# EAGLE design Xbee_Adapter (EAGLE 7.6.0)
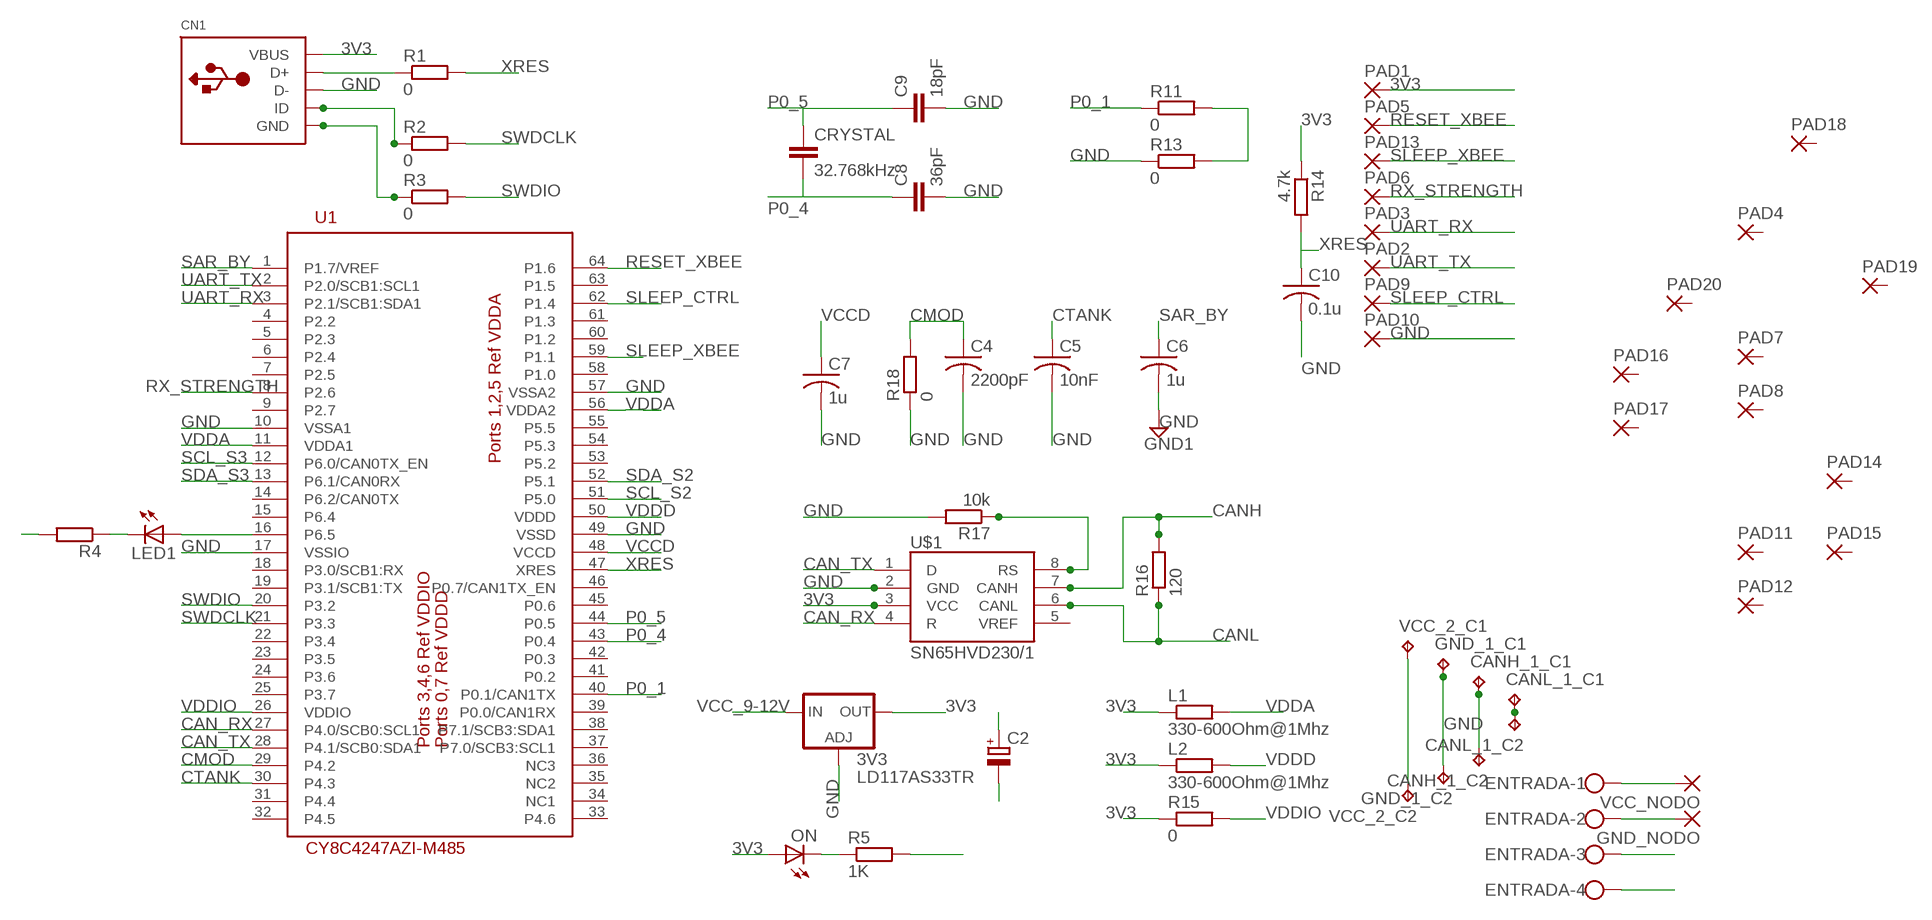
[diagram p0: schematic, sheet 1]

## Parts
3V3  LD117AS33TR  [SOT223]
C2  CPOL-EUA  [PANASONIC_A]
C4  2200pF  C-USC0805  [C0805]
C5  10nF  C-USC0805  [C0805]
C6  1u  C-USC0805  [C0805]
C7  1u  C-USC0805  [C0805]
C8  36pF  C-EUC0805  [C0805]
C9  18pF  C-EUC0805  [C0805]
C10  0.1u  C-USC0805  [C0805]
CANH_1_C1  TPB2,54  [B2,54]
CANH_1_C2  TPB2,54  [B2,54]
CANL_1_C1  TPB2,54  [B2,54]
CANL_1_C2  TPB2,54  [B2,54]
CN1  USBMINIB  [USB-MINIB]
CRYSTAL  32.768kHz  C-EUC0603  [C0603]
ENTRADA  W237-4  [W237-4]
GND_1_C1  TPB2,54  [B2,54]
GND_1_C2  TPB2,54  [B2,54]
GND_NODO  SMD5  [SMD2,54-5,08]
L1  330-600Ohm@1Mhz  R-EU_R0805  [R0805]
L2  330-600Ohm@1Mhz  R-EU_R0805  [R0805]
LED1  LEDCHIP-LED0805  [CHIP-LED0805]
ON  LEDCHIP-LED0805  [CHIP-LED0805]
PAD1  SMD5  [SMD2,54-5,08]
PAD2  SMD5  [SMD2,54-5,08]
PAD3  SMD5  [SMD2,54-5,08]
PAD4  SMD5  [SMD2,54-5,08]
PAD5  SMD5  [SMD2,54-5,08]
PAD6  SMD5  [SMD2,54-5,08]
PAD7  SMD5  [SMD2,54-5,08]
PAD8  SMD5  [SMD2,54-5,08]
PAD9  SMD5  [SMD2,54-5,08]
PAD10  SMD5  [SMD2,54-5,08]
PAD11  SMD5  [SMD2,54-5,08]
PAD12  SMD5  [SMD2,54-5,08]
PAD13  SMD5  [SMD2,54-5,08]
PAD14  SMD5  [SMD2,54-5,08]
PAD15  SMD5  [SMD2,54-5,08]
PAD16  SMD5  [SMD2,54-5,08]
PAD17  SMD5  [SMD2,54-5,08]
PAD18  SMD5  [SMD2,54-5,08]
PAD19  SMD5  [SMD2,54-5,08]
PAD20  SMD5  [SMD2,54-5,08]
R1  0  R-EU_R0805  [R0805]
R2  0  R-EU_R0805  [R0805]
R3  0  R-EU_R0805  [R0805]
R4  R-EU_R0805  [R0805]
R5  1K  R-EU_R0805  [R0805]
R11  0  R-EU_R0805  [R0805]
R13  0  R-EU_R0805  [R0805]
R14  4.7k  R-EU_R0805  [R0805]
R15  0  R-EU_R0805  [R0805]
R16  120  R-EU_R0805  [R0805]
R17  10k  R-EU_R0805  [R0805]
R18  0  R-EU_R0805  [R0805]
U1  CY8C4247AZI-M485  [TQFP64-10X10]
U$1  SN65HVD230/1  [SO8]
VCC_2_C1  TPB2,54  [B2,54]
VCC_2_C2  TPB2,54  [B2,54]
VCC_NODO  SMD5  [SMD2,54-5,08]

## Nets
3V3: 3V3.4(OUT) C2.+ CN1.VBUS L1.1 L2.1 ON.A PAD1.1(P) R14.1 R15.1 U$1.3(VCC)
CAN_RX: U1.27(P4.0/SCB0:SCL1) U$1.4(R)
CAN_TX: U1.28(P4.1/SCB0:SDA1) U$1.1(D)
CANH: CANH_1_C1.TP CANH_1_C2.TP ENTRADA.3 R16.2 U$1.7(CANH)
CANL: CANL_1_C1.TP CANL_1_C2.TP ENTRADA.4 R16.1 U$1.6(CANL)
CMOD: C4.1 R18.2 U1.29(P4.2)
CTANK: C5.1 U1.30(P4.3)
GND: 3V3.1(ADJ) C2.- C4.2 C5.2 C6.2 C7.2 C8.2 C9.2 C10.2 CN1.D- ENTRADA.2 GND_1_C1.TP GND_1_C2.TP GND_NODO.1(P) PAD10.1(P) R4.2 R5.2 R13.1 R17.2 R18.1 U1.10(VSSA1) U1.17(VSSIO) U1.49(VSSD) U1.57(VSSA2) U$1.2(GND) ; supply symbol labelled GND1
N$1: CN1.D+ R1.1
N$2: CN1.ID R2.1
N$3: CN1.GND R3.1
N$4: R11.2 R13.2
N$5: LED1.A U1.16(P6.5)
N$6: LED1.C R4.1
N$9: R17.1 U$1.8(RS)
N$10: ON.C R5.1
P0_1: R11.1 U1.40(P0.1/CAN1TX)
P0_4: C8.1 CRYSTAL.2 U1.43(P0.4)
P0_5: C9.1 CRYSTAL.1 U1.44(P0.5)
RESET_XBEE: PAD5.1(P) U1.64(P1.6)
RX_STRENGTH: PAD6.1(P) U1.8(P2.6)
SAR_BY: C6.1 U1.1(P1.7/VREF)
SCL_S2: U1.51(P5.0)
SCL_S3: U1.12(P6.0/CAN0TX_EN)
SDA_S2: U1.52(P5.1)
SDA_S3: U1.13(P6.1/CAN0RX)
SLEEP_CTRL: PAD9.1(P) U1.62(P1.4)
SLEEP_XBEE: PAD13.1(P) U1.59(P1.1)
SWDCLK: R2.2 U1.21(P3.3)
SWDIO: R3.2 U1.20(P3.2)
UART_RX: PAD3.1(P) U1.3(P2.1/SCB1:SDA1)
UART_TX: PAD2.1(P) U1.2(P2.0/SCB1:SCL1)
VCC_9-12V: 3V3.3(IN) ENTRADA.1 VCC_2_C1.TP VCC_2_C2.TP VCC_NODO.1(P)
VCCD: C7.1 U1.48(VCCD)
VDDA: L1.2 U1.11(VDDA1) U1.56(VDDA2)
VDDD: L2.2 U1.50(VDDD)
VDDIO: R15.2 U1.26(VDDIO)
XRES: C10.1 R1.2 R14.2 U1.47(XRES)
Unconnected: PAD4.1(P) PAD7.1(P) PAD8.1(P) PAD11.1(P) PAD12.1(P) PAD14.1(P) PAD15.1(P) PAD16.1(P) PAD17.1(P) PAD18.1(P) PAD19.1(P) PAD20.1(P) U1.4(P2.2) U1.5(P2.3) U1.6(P2.4) U1.7(P2.5) U1.9(P2.7) U1.14(P6.2/CAN0TX) U1.15(P6.4) U1.18(P3.0/SCB1:RX) U1.19(P3.1/SCB1:TX) U1.22(P3.4) U1.23(P3.5) U1.24(P3.6) U1.25(P3.7) U1.31(P4.4) U1.32(P4.5) U1.33(P4.6) U1.34(NC1) U1.35(NC2) U1.36(NC3) U1.37(P7.0/SCB3:SCL1) U1.38(P7.1/SCB3:SDA1) U1.39(P0.0/CAN1RX) U1.41(P0.2) U1.42(P0.3) U1.45(P0.6) U1.46(P0.7/CAN1TX_EN) U1.53(P5.2) U1.54(P5.3) U1.55(P5.5) U1.58(P1.0) U1.60(P1.2) U1.61(P1.3) U1.63(P1.5) U$1.5(VREF)

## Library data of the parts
3V3 = v-reg:LD117A?*: Low drop fixed and adjustable positive voltage regulators 1 A Source: http://www.st.com/stonline/products/literature/ds/7194/ld1117axx.pdf
C2 = rcl:CPOL-EU: POLARIZED CAPACITOR, European symbol
C4-C7 C10 = rcl:C-US: CAPACITOR, American symbol
C8 C9 CRYSTAL = rcl:C-EU: CAPACITOR, European symbol
CANH_1_C1 CANH_1_C2 CANL_1_C1 CANL_1_C2 GND_1_C1 GND_1_C2 VCC_2_C1 VCC_2_C2 = testpad:TP: Test pad
CN1 = adafruit:USB: USB Connectors USBMINIB - Surface Mount Female Mini-B USB Connector 4UConnector: 06564 By microbuilder.eu Thru-hole RA Female Mini-B USB Connector 4UConnector: 18732 By ladyada.net
ENTRADA = con-wago-500:W237-4: WAGO SCREW CLAMP; OC_FARNELL: unknown; OC_NEWARK: unknown
GND_NODO PAD1-PAD20 VCC_NODO = wirepad:SMD5: SMD PAD
L1 L2 R1-R5 R11 R13-R18 = rcl:R-EU_: RESISTOR, European symbol
LED1 ON = adafruit:LED: LED
U1 = CypressPSoC:CY8C4247AZI-M485
U$1 = texas_instruments:SN65HVD230/1

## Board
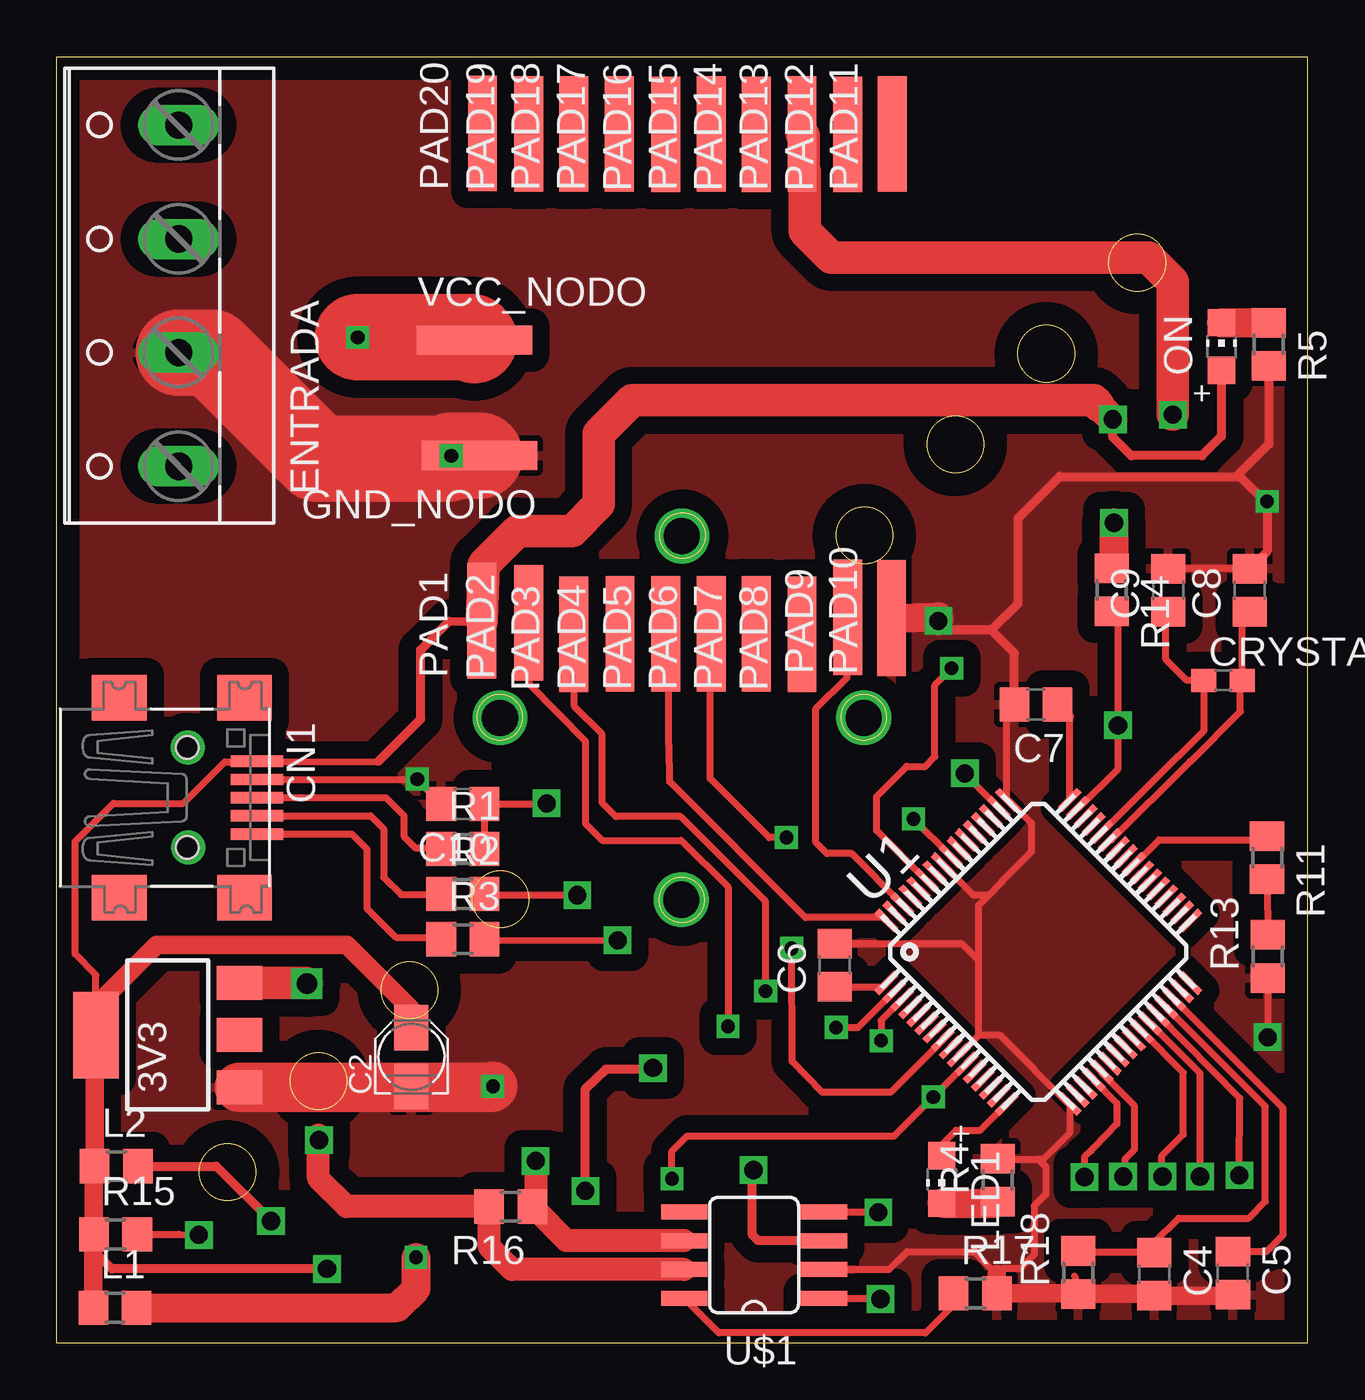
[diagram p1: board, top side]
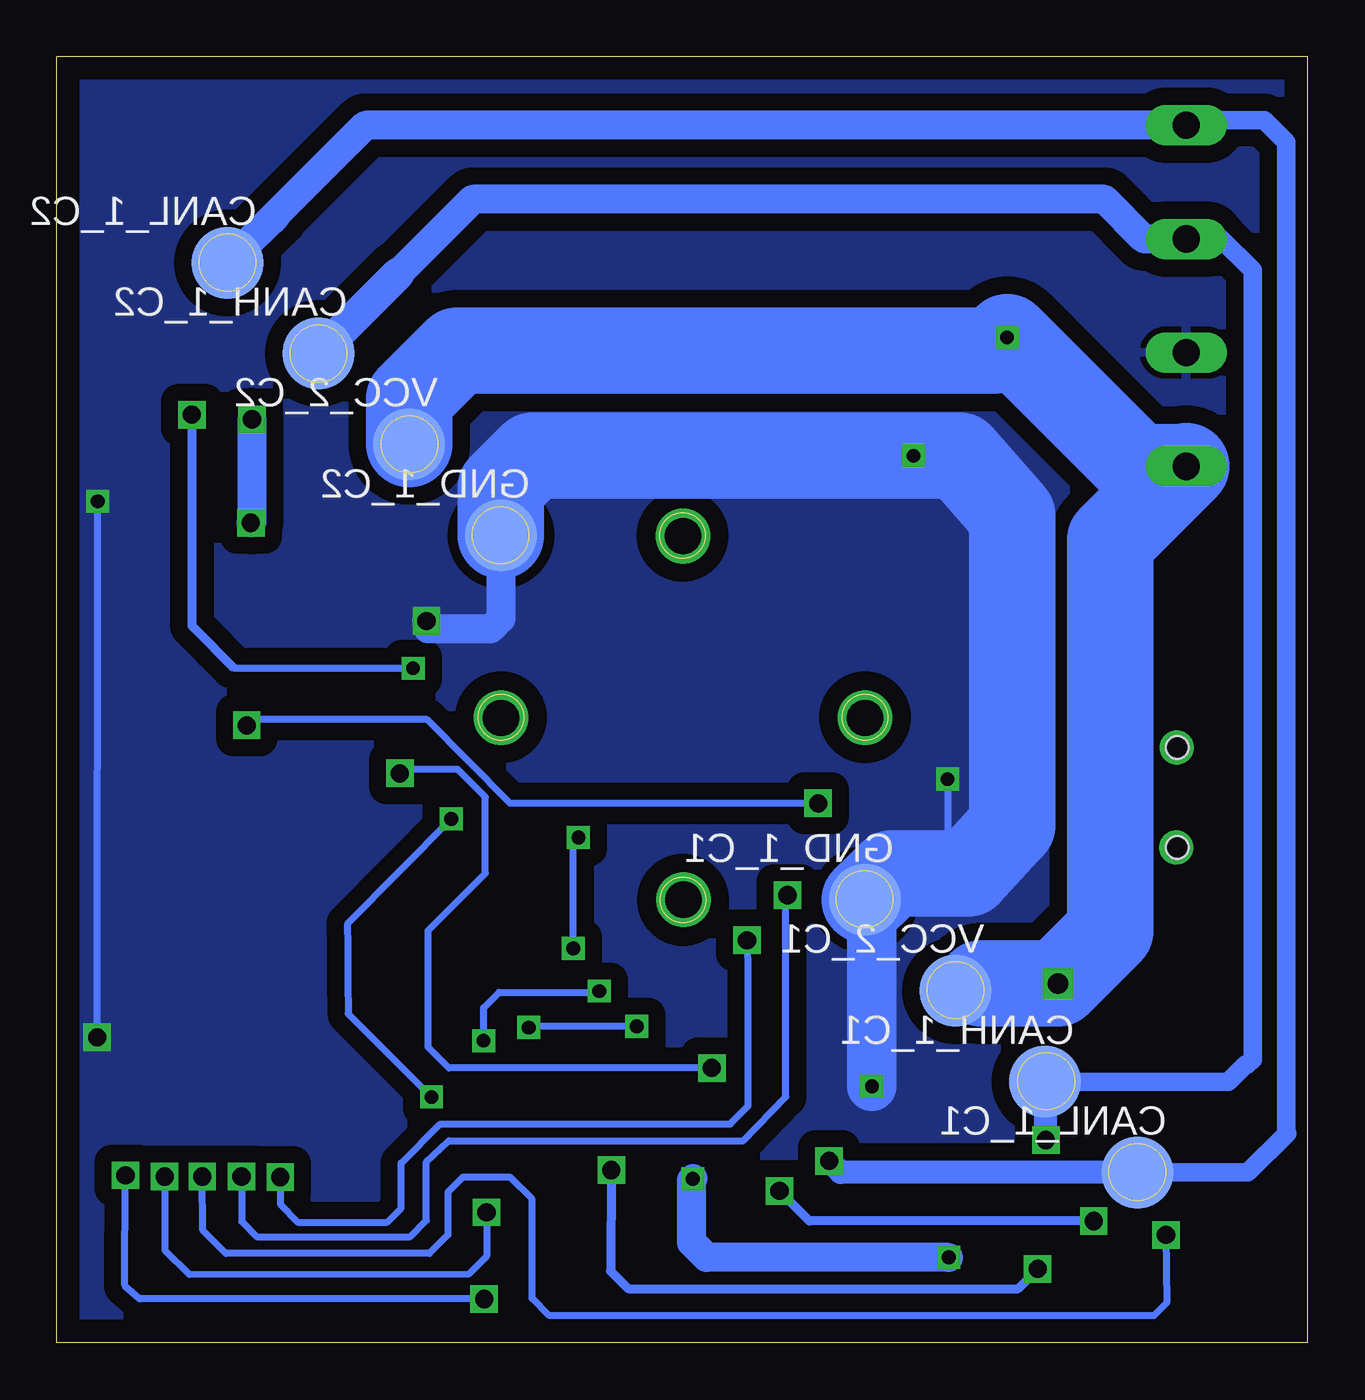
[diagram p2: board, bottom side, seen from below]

Size 55 x 56.55 mm. Coordinates in mm from the lower left corner, seen from the top.
Outline: 0,0 0,56.55 55,56.55 55,0 0,0
Outline: circle at 27.47,19.47 radius 1
Outline: circle at 19.47,27.5 radius 1
Outline: circle at 35.47,27.5 radius 1
Outline: circle at 43.5,43.5 radius 1.25
Outline: circle at 47.5,47.5 radius 1.25
Outline: circle at 43.5,43.5 radius 1.25
Outline: circle at 39.5,39.5 radius 1.25
Outline: circle at 35.5,35.5 radius 1.25
Outline: circle at 15.5,15.5 radius 1.25
Outline: circle at 11.5,11.5 radius 1.25
Outline: circle at 47.5,47.5 radius 1.25
Outline: circle at 39.5,39.5 radius 1.25
Outline: circle at 19.5,19.5 radius 1.25
Outline: circle at 7.5,7.5 radius 1.25
Outline: circle at 19.5,19.5 radius 1.25
Outline: circle at 15.5,15.5 radius 1.25
Outline: circle at 11.5,11.5 radius 1.25
Outline: circle at 35.5,35.5 radius 1.25
Outline: circle at 27.5,35.5 radius 1
Outline: circle at 7.5,7.5 radius 1.25
Copper layers (1*16): Top 0.035mm / dielectric 1.5mm / Bottom 0.035mm
Design rules "default": minimum track width 10mil, minimum drill 24mil, track to track 8mil, track to pad 8mil, pad to pad 8mil, via to via 8mil, smd to smd 8mil, copper to edge 40mil, drill to drill 8mil, minimum pad ring 10mil, minimum via ring 8mil, stop-mask expansion 4mil, vias tented up to drill 0mil, thermal gap 10mil

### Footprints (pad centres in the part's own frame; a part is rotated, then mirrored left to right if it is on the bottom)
SOT223 = smd 1.5 x 2: 1 -2.3,-3.15; 2 0,-3.15; 3 2.3,-3.15 | smd 3.8 x 2: 4 0,3.15
PANASONIC_A = smd 2 x 1.5: + 1.3,0; - -1.3,0
C0805 = smd 1.3 x 1.5: 1 -0.95,0; 2 0.95,0
B2,54 = smd 3.175 x 3.175 bottom: P$1 0,0 | smd 2.54 x 2.54 bottom: TP 0,0
USB-MINIB = smd 0.5 x 2.308: D+ 0,4.064; D- -0.8,4.064; GND 1.6,4.064; ID 0.8,4.064; VBUS -1.6,4.064 | smd 2 x 2.4: GND1 -4.4,-2; GND2 -4.4,3.5; GND3 4.4,3.5; GND4 4.4,-2 | hole 1: -2.2,1; 2.2,1
C0603 = smd 1.1 x 1: 1 -0.85,0; 2 0.85,0
W237-4 = drill 1.194 long: 1 -7.5,-1.27; 2 -2.5,-1.27; 3 2.5,-1.27; 4 7.5,-1.27
SMD2,54-5,08 = smd 1.27 x 5.08: 1 0,0
R0805 = smd 1.3 x 1.5: 1 -0.95,0; 2 0.95,0
CHIP-LED0805 = smd 1.2 x 1.2: A 0,-1.05; C 0,1.05
TQFP64-10X10 = smd 1.2 x 0.3: 1 -5.7,3.75; 2 -5.7,3.25; 3 -5.7,2.75; 4 -5.7,2.25; 5 -5.7,1.75; 6 -5.7,1.25; 7 -5.7,0.75; 8 -5.7,0.25; 9 -5.7,-0.25; 10 -5.7,-0.75; 11 -5.7,-1.25; 12 -5.7,-1.75; 13 -5.7,-2.25; 14 -5.7,-2.75; 15 -5.7,-3.25; 16 -5.7,-3.75; 33 5.7,-3.75; 34 5.7,-3.25; 35 5.7,-2.75; 36 5.7,-2.25; 37 5.7,-1.75; 38 5.7,-1.25; 39 5.7,-0.75; 40 5.7,-0.25; 41 5.7,0.25; 42 5.7,0.75; 43 5.7,1.25; 44 5.7,1.75; 45 5.7,2.25; 46 5.7,2.75; 47 5.7,3.25; 48 5.7,3.75 | smd 0.3 x 1.2: 17 -3.75,-5.7; 18 -3.25,-5.7; 19 -2.75,-5.7; 20 -2.25,-5.7; 21 -1.75,-5.7; 22 -1.25,-5.7; 23 -0.75,-5.7; 24 -0.25,-5.7; 25 0.25,-5.7; 26 0.75,-5.7; 27 1.25,-5.7; 28 1.75,-5.7; 29 2.25,-5.7; 30 2.75,-5.7; 31 3.25,-5.7; 32 3.75,-5.7; 49 3.75,5.7; 50 3.25,5.7; 51 2.75,5.7; 52 2.25,5.7; 53 1.75,5.7; 54 1.25,5.7; 55 0.75,5.7; 56 0.25,5.7; 57 -0.25,5.7; 58 -0.75,5.7; 59 -1.25,5.7; 60 -1.75,5.7; 61 -2.25,5.7; 62 -2.75,5.7; 63 -3.25,5.7; 64 -3.75,5.7
SO8 = smd 0.66 x 2.032: 1 -1.905,-3.073; 2 -0.635,-3.073; 3 0.635,-3.073; 4 1.905,-3.073; 5 1.905,3.073; 6 0.635,3.073; 7 -0.635,3.073; 8 -1.905,3.073

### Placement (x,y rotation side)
3V3  4.87,13.53 90 top
C2  15.59,12.56 90 top
C4  48.25,3.01 270 top
C5  51.71,3.07 270 top
C6  34.21,16.6 90 top
C7  43.04,28.06 180 top
C8  52.44,33.09 90 top
C9  48.86,33.09 90 top
C10  17.85,23.69 180 top
CANH_1_C1  11.55,11.47 0 top
CANH_1_C2  43.5,43.5 0 top
CANL_1_C1  7.48,7.48 0 top
CANL_1_C2  47.49,47.49 0 top
CN1  4.74,23.97 270 top
CRYSTAL  51.27,29.13 0 top
ENTRADA  4.08,46.04 90 top
GND_1_C1  19.47,19.47 0 top
GND_1_C2  35.48,35.5 0 top
GND_NODO  18.58,39.01 90 top
L1  2.56,1.54 0 top
L2  2.61,7.76 0 top
LED1  38.9,7.18 180 top
ON  51.2,43.81 0 top
PAD1  18.69,31.74 0 top
PAD2  20.74,31.67 0 top
PAD3  22.72,31.16 0 top
PAD4  24.76,31.18 0 top
PAD5  26.76,31.18 0 top
PAD6  28.77,31.18 0 top
PAD7  30.75,31.18 0 top
PAD8  32.76,31.16 0 top
PAD9  34.76,31.89 0 top
PAD10  36.69,31.87 0 top
PAD11  36.72,53.15 0 top
PAD12  34.76,53.13 0 top
PAD13  32.76,53.15 0 top
PAD14  30.75,53.13 0 top
PAD15  28.77,53.15 0 top
PAD16  26.76,53.13 0 top
PAD17  24.73,53.15 0 top
PAD18  22.72,53.15 0 top
PAD19  20.74,53.15 0 top
PAD20  18.71,53.18 0 top
R1  17.85,21.71 0 top
R2  17.85,19.73 0 top
R3  17.85,17.75 0 top
R4  41.37,7.15 90 top
R5  53.28,43.91 270 top
R11  53.2,21.33 270 top
R13  53.23,16.98 90 top
R14  46.37,33.11 270 top
R15  2.58,4.77 0 top
R16  19.96,5.99 180 top
R17  40.38,2.18 0 top
R18  44.9,3.09 90 top
U1  43.15,17.19 45 top
U$1  30.65,3.85 90 top
VCC_2_C1  15.49,15.49 0 top
VCC_2_C2  39.51,39.51 0 top
VCC_NODO  18.36,44.09 270 top

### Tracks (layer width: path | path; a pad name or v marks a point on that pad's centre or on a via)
3V3  (via drill 0.8)
  Top 0.305: 3V3.4 1.72,14.8 1.72,16.17 0.8,17.09 0.8,22.04 2.48,23.72 5.55,23.72 7.38,25.54 8.78,25.54 CN1.VBUS 14.06,25.54 15.99,27.45
  Top 0.406: U$1.3 30.83,4.49 30.57,4.74 30.57,7.71 v30.62,7.59 | v11.88,3.24 2.42,3.24 1.61,4.06 | PAD1.1 17.24,31.72 15.99,30.47 15.99,27.45 15.99,27.42 14.14,25.57 | ON.A 51.2,39.87 50.33,39.01 47.24,39.01 46.42,39.82 v46.42,40.61
  Top 0.813: L1.1 1.61,4.06 1.61,4.74 R15.1 1.63,7.74 L2.1 1.66,13.47 3V3.4 | C2.+ 15.59,14.65 12.74,17.49 4.39,17.49 1.72,14.8
  Top 1.27: 45.81,41.22 v46.42,40.61 | v46.47,36.06 46.47,34.16 R14.1
  Top 1.422: PAD1.1 18.76,34.23 20.24,35.7 22.65,35.7 23.82,36.87 23.82,39.97 25.29,41.44 45.58,41.44 45.81,41.22
  Bottom 0.406: v30.62,7.59 30.65,3.14 29.89,2.38 12.74,2.38 v11.88,3.24
  Bottom 1.27: v46.42,40.61 46.42,36.11 v46.47,36.06
CAN_RX  (via drill 0.8)
  Top 0.305: U$1.4 36.09,5.76 v36.11,5.73 | v50.26,7.31 50.26,11.84 U1.27
  Bottom 0.305: v36.11,5.73 36.11,3.8 36.9,3.01 49.17,2.99 50.23,4.03 50.23,7.28 v50.26,7.31
CAN_TX  (via drill 0.8)
  Top 0.305: U$1.1 36.19,1.95 v36.21,1.92 | v51.99,7.36 52.01,10.75 U1.28
  Bottom 0.305: v36.21,1.92 51.35,1.92 52.01,2.51 v51.99,7.36
CANH  (via drill 0.8)
  Top 1.016: U$1.7 20.01,3.22 19.02,4.21 19.02,5.98 R16.2 12.74,5.99 11.5,7.23 11.5,9.14 v11.52,8.91
  Bottom 0.813: CANH_1_C1.TP 3.5,11.47 2.73,12.23 2.63,12.23 2.43,12.44 2.43,47.16 3.85,48.58 5.31,48.58
  Bottom 1.016: v11.52,8.91 11.52,11.45 CANH_1_C1.TP
  Bottom 1.27: 42.89,44.11 CANH_1_C2.TP | 5.31,48.58 ENTRADA.3 7.19,48.54 8.93,50.28 36.72,50.28 40.75,46.26
  Bottom 1.422: 40,47.01 40.75,46.26 42.89,44.11
CANL  (via drill 0.8)
  Top 1.016: U$1.6 22.4,4.49 21.05,5.84 | 21.05,5.84 R16.1 | v21.05,7.99 21.05,5.84
  Bottom 0.813: CANL_1_C1.TP 2.63,7.48 0.91,9.21 0.96,9.21 0.96,52.8 1.92,53.76 5.13,53.76
  Bottom 1.016: CANL_1_C1.TP 20.54,7.48 v21.05,7.99
  Bottom 1.27: 45.36,49.55 CANL_1_C2.TP 41.44,53.54 ENTRADA.4 5.13,53.76
CMOD
  Top 0.305: R18.2 44.98,3.96 C4.1 48.25,4.41 49.32,5.48 52.39,5.48 53.13,6.21 53.13,10.39 U1.29 48.81,14.75
CTANK
  Top 0.305: C5.1 53.19,4.02 53.92,4.74 53.92,10.31 U1.30
GND  (via drill 0.6, 0.8)
  Top 0.305: 44.75,2.93 R18.1 | U$1.2 36.59,3.22 37.38,4 40.34,4 41.33,3.01 41.56,3.24 42.33,3.24 42.97,3.88 42.97,6.01 43.48,6.52 43.48,7.74 43.15,8.07 | CN1.D- 15.82,24.77 C10.2 16.9,23.73 v15.84,24.78 | C9.2 C8.2 53.26,34.85 | R13.1 v53.23,13.43 | 38.78,31.44 v38.75,31.74 | 40.52,13.5 41.47,13.5 44.47,10.51 U1.17 44.53,9.22 43.37,8.07 43.15,8.07 | 40.52,13.5 U1.10 | 41.77,27.73 U1.49 41.82,23.87 42.84,22.85 42.84,21.58 41.52,20.26 41.52,20.24 40.96,19.68 | 40.96,19.68 40.3,19.68 U1.57 | 40.52,13.5 40.52,16.81 | 40.52,16.81 40.52,19.24 40.96,19.68 | C6.2 39.78,17.55 40.52,16.81 | R4.2 41.4,8.07 43.15,8.07 | C2.- 7.9,11.26 7.87,11.29 7.97,11.29 8.07,11.19
  Top 0.406: 41.09,31.34 42.09,30.33 C7.2 41.77,27.73 | 41.09,31.34 38.83,31.34 v38.75,31.74 | 41.09,31.34 42.26,32.5 42.26,36.26 44.09,38.09 51.86,38.09 | 51.86,38.09 52.01,38.09 53.2,36.9 53.2,34.8 C8.2 53.2,34.8 v53.2,37 | R5.2 53.28,39.51 51.86,38.09
  Top 0.813: 41.33,3.01 R17.2 44.86,2.18 R18.1 48.18,2.14 C4.2 51.6,2.06 C5.2
  Top 1.27: PAD10.1 38.75,31.92 v38.75,31.74
  Top 2.184: 3V3.1 19.13,11.23 v19.17,11.27
  Top 3.81: GND_NODO.1 v17.34,39.01 17.21,38.88 11.47,38.88 6.81,43.54 ENTRADA.2
  Bottom 0.305: v53.23,13.43 v53.2,37 | v15.84,24.78 15.84,21.4 15.08,20.64
  Bottom 1.27: GND_1_C2.TP 35.48,31.84 35.93,31.39 38.68,31.39 v38.75,31.74
  Bottom 2.184: v19.17,11.27 19.17,19.78 18.97,19.98
  Bottom 3.81: 13.1,36.21 13,36.36 | 13,36.36 13,22.75 14.93,20.64 15.08,20.64 18.31,20.64 18.97,19.98 GND_1_C1.TP | GND_1_C2.TP 35.48,37.61 34.08,39.01 v17.34,39.01 15.31,39.01 13,36.36
  pour Bottom (isolate 0.762): -0.21,56.51 -0.24,24.4 -0.62,10.23 -0.59,10.33 -0.59,-0.24 54.65,-0.34 54.86,56.38 3.34,56.48
  pour Top (isolate 0.762): -0.74,56.53 -0.21,24.48 -0.36,24.53 -0.59,10.2 -0.62,10.23 -0.54,-0.36 54.65,-0.29 54.7,56.46
N$1
  Top 0.305: CN1.D+ 14.47,23.97 15.26,23.18 15.26,22.27 15.77,21.76 16.85,21.76 R1.1
N$2
  Top 0.305: CN1.ID 13.8,23.17 14.37,22.6 14.37,20.46 15.13,19.7 16.87,19.7 R2.1
N$3
  Top 0.305: CN1.GND 12.97,22.37 13.63,21.71 13.63,19.09 14.9,17.82 16.82,17.82 R3.1
N$4
  Top 0.305: R11.2 53.2,20.12 R13.2
N$5
  Top 0.305: LED1.A 38.9,8.7 39.54,9.34 40.6,9.34 U1.16
N$6
  Top 1.27: LED1.C 41.29,6.13 R4.1
N$7  (via drill 1)
  other vias: 5.76,26.18
N$8  (via drill 1)
  other vias: 5.78,21.79
N$9
  Top 0.305: R17.1 39.43,1.66 38.19,0.42 29.1,0.42 U$1.8
N$10
  Top 1.27: ON.C R5.1
N$23  (via drill 1.6)
  other vias: 35.48,27.47
N$24  (via drill 1.6)
  other vias: 27.47,35.48
N$25  (via drill 1.6)
  other vias: 19.47,27.47
N$28  (via drill 1.6)
  other vias: 27.45,19.47
P0_1
  Top 0.305: U1.40 47.38,21.04 48.45,22.12 53.04,22.12 R11.1
P0_4
  Top 0.305: C8.1 52.12,31.82 CRYSTAL.2 52.04,29.04 52.04,27.75 49.85,25.57 49.83,25.57 46.36,22.1 U1.43
P0_5
  Top 0.305: C9.1 48.76,32.04 48.76,30.04 49.67,29.13 CRYSTAL.1 50.44,29.11 50.44,26.92 49.32,25.8 49.29,25.8 45.95,22.46 U1.44
RESET_XBEE
  Top 0.305: U1.64 36.28,18.69 32.9,18.69 26.94,24.68 26.92,26.28 26.89,26.31 26.89,31.06 PAD5.1
RX_STRENGTH  (via drill 0.6)
  Top 0.305: U1.8 38.94,13.29 36.67,11.02 33.65,11.02 32.33,12.36 v32.3,17.34 | v32.07,22.22 31.31,22.22 28.72,24.81 28.72,31.13 PAD6.1
  Bottom 0.305: v32.3,17.34 32.3,21.99 v32.07,22.22
SAR_BY
  Top 0.305: C6.1 36.31,15.65 U1.1
SLEEP_CTRL
  Top 0.305: U1.62 34.94,21.51 33.85,21.51 33.37,21.99 33.37,27.88 34.74,29.25 34.74,31.39 PAD9.1
SLEEP_XBEE  (via drill 0.6, 0.8)
  Top 0.305: U1.59 38.22,20.33 36.03,22.52 36.03,24.02 37.36,25.34 38.17,25.34 38.6,25.77 38.6,28.92 v39.34,29.66
  Top 1.422: v49.06,40.81 49.06,46.65 48,47.72 34.05,47.72 32.88,48.89 32.88,51.53 32.83,51.58 32.83,53.08 PAD13.1
  Bottom 0.305: v39.34,29.66 47.21,29.66 47.29,29.74
  Bottom 0.406: v49.06,40.81 49.06,31.54 48.07,30.55 48.07,30.52 47.29,29.74
SWDCLK  (via drill 0.8)
  Top 0.305: U1.21 45.94,11.85 47.36,10.43 47.36,8.48 46.96,8.07 46.96,7.48 v46.88,7.31 | v22.88,19.68 18.85,19.68 R2.2
  Bottom 0.305: v46.88,7.31 46.88,5.33 46.22,4.67 39.46,4.67 38.75,5.38 38.75,7.94 37.76,8.88 24.83,8.88 22.95,10.81 22.95,19.22 v22.88,19.68
SWDIO  (via drill 0.8)
  Top 0.305: U1.20 45.59,11.55 46.6,10.53 46.6,9.62 45.56,8.55 45.48,8.45 45.18,8.17 v45.18,7.28 | v24.66,17.7 18.87,17.67 R3.2
  Bottom 0.305: v45.18,7.28 45.18,6.09 44.42,5.3 40.48,5.3 39.87,5.91 39.87,7.89 38.14,9.62 25.39,9.62 24.6,10.41 24.6,16.68 v24.66,17.7
UART_RX  (via drill 0.6)
  Top 0.305: U1.3 36.24,14.16 v36.24,13.28 | v31.16,15.46 31.16,19.4 27.42,23.13 24.58,23.13 23.97,23.74 23.97,26.76 22.75,27.98 22.75,31.13 PAD3.1
  Bottom 0.305: v36.24,13.28 36.24,14.72 35.55,15.41 31.21,15.41 v31.16,15.46
UART_TX  (via drill 0.6)
  Top 0.305: PAD2.1 20.74,29 23.23,26.46 23.23,22.83 23.97,22.09 27.45,22.09 29.51,20.03 v29.51,13.91 | v34.26,13.86 35.22,13.86 U1.2
  Bottom 0.305: v29.51,13.91 34.31,13.91 v34.26,13.86
VCC_9-12V  (via drill 0.6, 0.9)
  Top 1.422: 3V3.3 10.95,15.83 v10.99,15.79
  Top 3.81: v13.23,44.21 18.23,44.21 VCC_NODO.1
  Bottom 1.422: 14.37,15.79 15.23,14.93 15.23,15.23 VCC_2_C1.TP
  Bottom 3.81: 8.68,35.21 8.68,18.1 v10.99,15.79 14.37,15.79 | 8.68,35.21 ENTRADA.1 | 8.68,35.21 8.68,35.32 5.5,38.5 7.51,38.5 v13.23,44.21 13.81,43.63 37.41,43.63 39.51,41.52 VCC_2_C2.TP
VCCD
  Top 0.305: U1.48 44.53,27.53
  Top 0.406: 44.53,27.53 C7.1
VDDA  (via drill 0.6)
  Top 0.305: v27.04,7.21 27.04,8.42 27.7,9.08 36.81,9.08 v38.53,10.8 U1.11 | U1.56 v37.66,23.03
  Top 1.27: L1.2 14.95,1.54 15.79,2.38 v15.79,3.75
  Bottom 0.305: v37.66,23.03 42.23,18.41 42.21,17.44 42.21,15.92 42.2,14.47 v38.53,10.8
  Bottom 1.27: v15.79,3.75 26.43,3.75 27.09,4.41 27.09,7.15 v27.04,7.21
VDDD  (via drill 0.8)
  Top 0.305: 39.92,25.01 U1.50
  Top 0.406: L2.2 7,7.76 v9.42,5.35 | v23.23,6.67 23.23,11.17 24.15,12.03 26.15,12.03 v26.2,12.08 | v39.92,25.04 39.92,25.01
  Bottom 0.305: v26.2,12.08 37.76,12.08 38.68,13 38.68,18.13 36.16,20.64 36.16,23.99 37.38,25.21 39.74,25.21 v39.92,25.04
  Bottom 0.406: v9.42,5.35 21.91,5.35 v23.23,6.67
VDDIO  (via drill 0.8)
  Top 0.305: R15.2 5.38,4.77 v6.24,4.74 | v48.61,7.31 48.58,8.22 49.52,9.16 49.52,11.87 U1.26
  Bottom 0.305: v48.61,7.31 48.58,4.94 47.57,3.93 38.63,3.93 37.81,4.74 37.81,6.62 37.15,7.28 35.07,7.28 34.1,6.32 34.1,1.95 33.34,1.19 6.77,1.19 6.21,1.74 v6.24,4.74
XRES  (via drill 0.8)
  Top 0.305: R1.2 C10.1 21.58,23.69 v21.53,23.72 | R14.2 46.65,31.88 v46.65,27.14 46.65,25.24 44.93,23.52 U1.47
  Bottom 0.305: v21.53,23.72 35.07,23.72 38.73,27.4 46.4,27.4 v46.65,27.14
